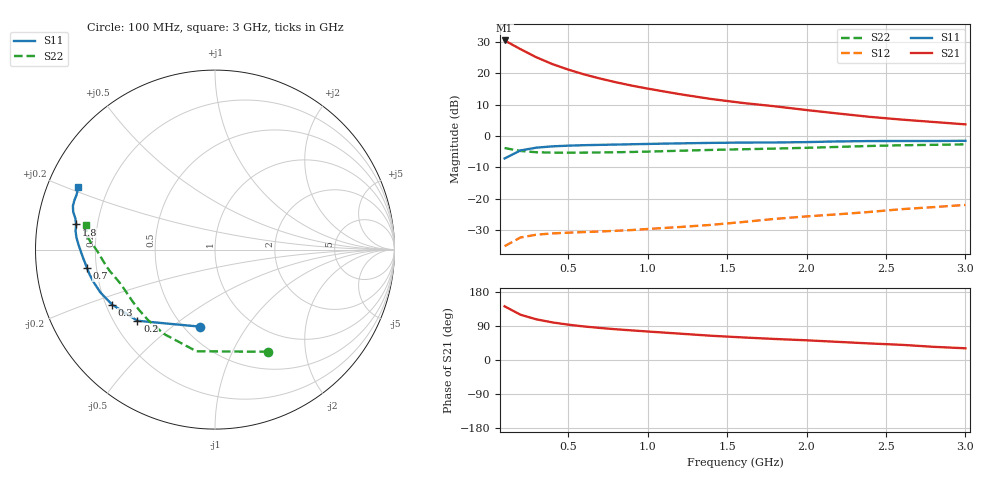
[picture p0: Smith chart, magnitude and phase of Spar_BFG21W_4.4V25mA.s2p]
! Filename: 4_425bfg21.001
! Title: BFG21W
! Bias: Vce=4.4V; Ic=25mA
! Company: NXP Semiconductors NL
! User: Quality&Reliability T&D
! Measure time: 10 Nov 1999 / 11:46:23
#  MHz  S  MA  R 50
! Freq  S11  S21  S12  S22  :
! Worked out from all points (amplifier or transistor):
!   20 points, 100 MHz to 3 GHz, reference 50 ohm
!   highest |S21| = 30.5 dB at 100 MHz (marker M1)
!   |S21| within 3 dB of that: start of sweep to 208.6 MHz
!   unconditionally stable (mu >= 1): 1.101 GHz to end of sweep
!   at 400 MHz: K = 0.50, MSG = 27.0 dB, |S12| = -31.1 dB
!   at 1.2 GHz: K = 1.04, MAG = 19.9 dB, |S12| = -29.1 dB
!   at 3 GHz: K = 1.04, MAG = 11.6 dB, |S12| = -22.0 dB
!   S11 on the Smith chart (normalised r, x): 100 MHz: 0.59, -0.63; 200 MHz: 0.30, -0.36; 300 MHz: 0.22, -0.24; 700 MHz: 0.16, -0.07; 1.8 GHz: 0.12, +0.09; 3 GHz: 0.09, +0.22
100  0.4374 -101.1  33.34 141.7  0.01744 42.6  0.6414 -62.5
200  0.5867 -137.5  24.22 119.5  0.02401 34.0  0.5759 -100.3
300  0.65 -151.9  17.96 107.3  0.02659 30.0  0.5493 -121.2
400  0.6818 -159.5  14.02 99.3  0.02786 29.2  0.5416 -133.7
500  0.6998 -164.9  11.45 93.3  0.02863 29.7  0.5405 -141.8
600  0.7122 -168.7  9.595 88.5  0.02928 31.3  0.5422 -147.5
700  0.7202 -171.7  8.241 84.6  0.02992 33.5  0.5451 -151.7
800  0.7279 -174.2  7.187 81.1  0.03068 36.1  0.5491 -155.2
900  0.7367 -176.5  6.351 78.1  0.03154 39.2  0.555 -158.1
1000  0.7452 -178.6  5.689 75.2  0.03279 42.0  0.5623 -160.8
1200  0.7611 177.9  4.644 69.6  0.03519 47.3  0.5802 -165.1
1400  0.7746 175.1  3.881 64.0  0.03814 52.0  0.5984 -168.5
1600  0.7834 172.5  3.354 59.5  0.04236 56.4  0.6132 -171.5
1800  0.7864 169.7  2.97 55.5  0.04748 60.1  0.6285 -174.6
2000  0.7971 167.4  2.59 52.0  0.05206 63.4  0.6465 -177.9
2200  0.8176 165.1  2.277 47.8  0.05628 65.3  0.6685 179.2
2400  0.8283 162.9  2.013 43.6  0.0614 66.4  0.6921 176.8
2600  0.8302 160.7  1.821 40.0  0.06794 67.0  0.71 174.7
2800  0.8296 158.2  1.668 34.8  0.07324 66.4  0.7215 172.3
3000  0.8369 155.5  1.53 30.9  0.07934 66.4  0.7338 169.4
